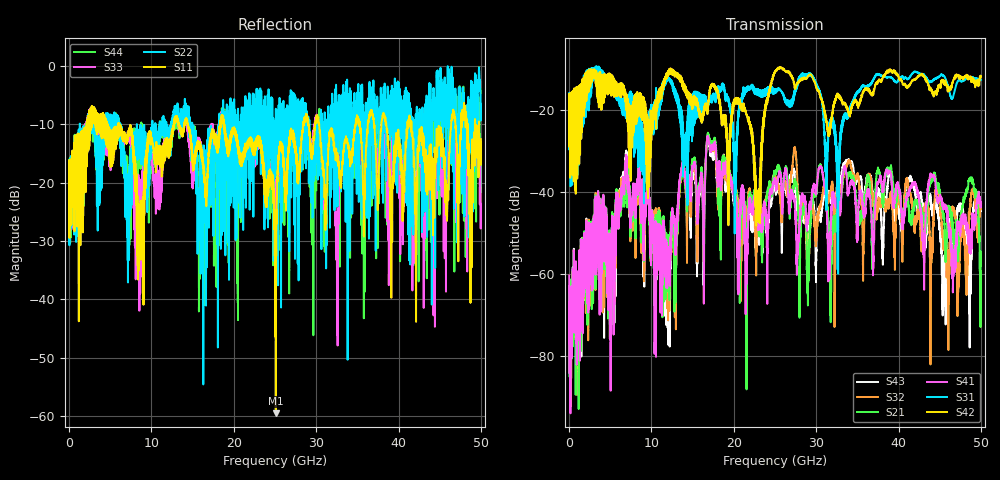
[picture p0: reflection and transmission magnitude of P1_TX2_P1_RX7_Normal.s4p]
!Keysight Technologies,N5225B,MY57041031,A.13.20.10
!Date: Friday, May 31, 2019 11:24:00
!Correction: S11(Full 4 Port(1,2,3,4))
!S12(Full 4 Port(1,2,3,4))
!S13(Full 4 Port(1,2,3,4))
!S14(Full 4 Port(1,2,3,4))
!S21(Full 4 Port(1,2,3,4))
!S22(Full 4 Port(1,2,3,4))
!S23(Full 4 Port(1,2,3,4))
!S24(Full 4 Port(1,2,3,4))
!S31(Full 4 Port(1,2,3,4))
!S32(Full 4 Port(1,2,3,4))
!S33(Full 4 Port(1,2,3,4))
!S34(Full 4 Port(1,2,3,4))
!S41(Full 4 Port(1,2,3,4))
!S42(Full 4 Port(1,2,3,4))
!S43(Full 4 Port(1,2,3,4))
!S44(Full 4 Port(1,2,3,4))
!S4P File: Measurements: <S11,S12,S13,S14>,
!<S21,S22,S23,S24>,
!<S31,S32,S33,S34>,
!<S41,S42,S43,S44>:
# Hz S  dB  R 50.0
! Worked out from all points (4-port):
!   5000 points, 10 MHz to 50 GHz, reference 50 ohm
!   strongest paths, dB at 10 MHz, 12.51 GHz, 25.01 GHz, 37.51 GHz, 50 GHz:
!     S42: -19.6, -10.0, -10.7, -12.8, -11.7
!     S31: -19.4, -13.0, -15.4, -11.1, -12.5
!     S41: -60.4, -45.0, -37.9, -37.8, -43.6
!     S21: -65.1, -45.2, -35.6, -34.3, -54.5
!     S32: -65.4, -47.1, -36.4, -42.4, -42.8
!     S43: -62.9, -46.4, -39.4, -39.2, -43.8
!   lowest |S11| = -59.6 dB at 25.1 GHz (marker M1), VSWR 1.00, Z = 49.9 + j0.0403 ohm
!   |S11| at or under -10 dB: 6.091 GHz to 12.71 GHz (6.616 GHz wide, 70.4 % of centre); 18.82 GHz to 28.43 GHz (9.603 GHz wide, 40.6 % of centre); 41.58 GHz to 46.39 GHz (4.81 GHz wide, 10.9 % of centre)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
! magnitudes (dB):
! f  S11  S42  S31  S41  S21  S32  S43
! 10 MHz  -19.9  -19.6  -19.4  -60.4  -65.1  -65.4  -62.9
! 6.8 GHz  -12.8  -17.6  -21.3  -35.1  -37.6  -35.5  -33.3
! 12.02 GHz  -12.6  -10.4  -12.1  -54.7  -53.2  -58.7  -65.3
! 16.88 GHz  -16.4  -18.5  -18.9  -26.3  -25.6  -25.8  -26.5
! 22.93 GHz  -12.0  -39.7  -16.0  -47.4  -47.6  -47.3  -49.7
! 25.1 GHz  -59.6  -10.4  -15.0  -39.5  -35.3  -36.9  -40.6
! 50 GHz  -12.6  -11.7  -12.5  -43.6  -54.5  -42.8  -43.8
